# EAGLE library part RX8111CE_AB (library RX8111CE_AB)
Real Time Clock RX8111CE:AB REAL TIME CLOCK I2C-BUS 3.0V 11.5PPM BULK Source: Datasheet
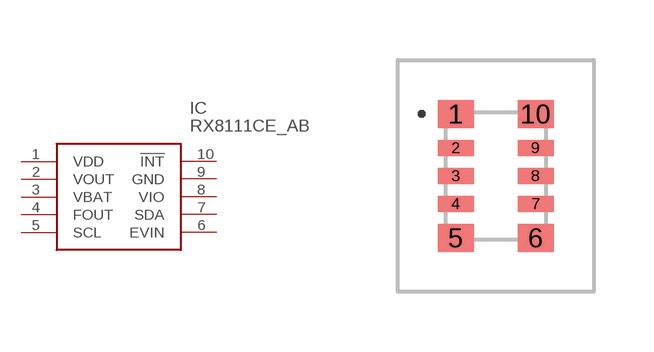
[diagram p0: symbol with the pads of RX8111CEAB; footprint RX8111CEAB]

Designator prefix IC

## RX8111CE_AB (Description: Real Time Clock RX8111CE:AB REAL TIME CLOCK I2C-BUS 3.0V 11.5PPM BULK; Height: 1mm; Manufacturer_Name: Epson Timing; Manufacturer_Part_Number: RX8111CE AB; Mouser_Part_Number: 732-RX8111CEAB; Mouser_Price-Stock: https://www.mouser.co.uk/ProductDetail/Epson-Timing/RX8111CE-AB?qs=zW32dvEIR3tJmkMUq44aCA%3D%3D)  [RX8111CEAB]
1  VDD
2  VOUT
3  VBAT
4  FOUT
5  SCL
6  EVIN
7  SDA
8  VIO
9  GND
10  !INT

## Footprint RX8111CEAB (pad centres in mm)
RX8111CE AB-1
smd 0.9 x 0.7: 1 -1,1.55; 5 -1,-1.55; 6 1,-1.55; 10 1,1.55
smd 0.9 x 0.4: 2 -1,0.7; 3 -1,0; 4 -1,-0.7; 7 1,-0.7; 8 1,0; 9 1,0.7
